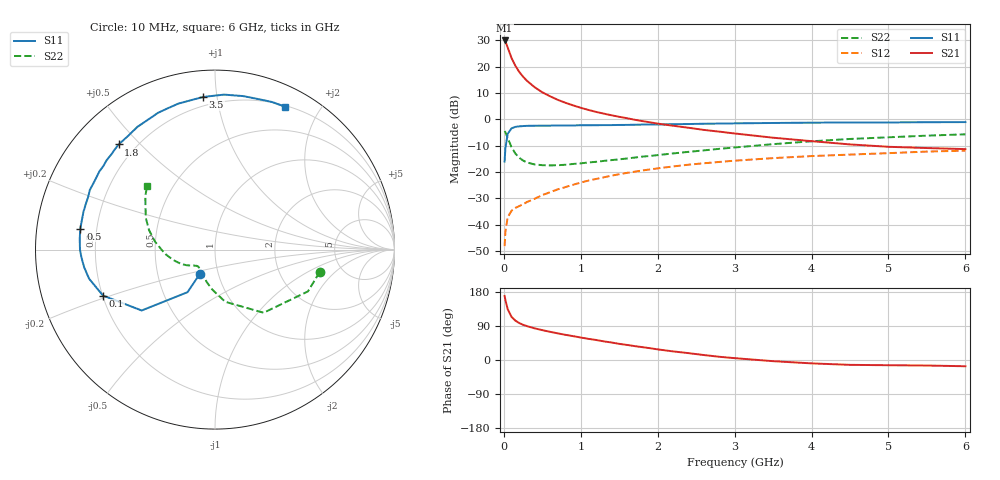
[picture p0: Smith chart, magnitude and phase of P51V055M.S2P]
! SIEMENS Small Signal Semiconductors
! BFP183
! Si NPN RF Bipolar Junction Transistor in SOT143
! VCE = 1 V  IC = 55 mA
! Common Emitter S-Parameters:  March  1996
# GHz  S  MA  R  50
!  f  S11  S21  S12  S22
! GHz  MAG  ANG  MAG  ANG  MAG  ANG  MAG  ANG
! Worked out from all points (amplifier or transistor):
!   36 points, 10 MHz to 6 GHz, reference 50 ohm
!   highest |S21| = 30.0 dB at 10 MHz (marker M1)
!   |S21| within 3 dB of that: start of sweep to 54.15 MHz
!   unconditionally stable (mu >= 1): start of sweep to 36.99 MHz; 132.7 MHz to end of sweep
!   at 250 MHz: K = 1.40, MAG = 20.5 dB, |S12| = -32.3 dB
!   at 1.4 GHz: K = 1.98, MAG = 5.8 dB, |S12| = -21.4 dB
!   at 6 GHz: K = 1.56, MAG = -4.1 dB, |S12| = -11.9 dB
!   S11 on the Smith chart (normalised r, x): 10 MHz: 0.82, -0.23; 100 MHz: 0.20, -0.19; 500 MHz: 0.14, +0.08; 1.8 GHz: 0.14, +0.43; 3.5 GHz: 0.15, +0.91; 6 GHz: 0.21, +1.58
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0.01  0.158 -121.9  31.5 169.0  0.0039 64.1  0.5965 -12.1
0.02  0.2823 -122.8  30.21 158.4  0.0074 60.8  0.5679 -24.2
0.05  0.5311 -140.3  23.17 134.2  0.0138 51.6  0.444 -52.4
0.1  0.6747 -157.7  14.62 113.9  0.0183 40.7  0.2963 -78.9
0.15  0.7202 -167.0  10.4 103.9  0.0208 40.5  0.2236 -93.8
0.2  0.7355 -172.3  7.962 97.5  0.0225 42.5  0.1868 -104.2
0.25  0.7457 -176.8  6.455 92.9  0.0244 45.0  0.1651 -111.7
0.3  0.7522 -179.9  5.407 89.4  0.0269 47.5  0.1517 -117.4
0.4  0.7562 175.4  4.076 83.6  0.031 52.5  0.1392 -125.5
0.5  0.7594 171.1  3.263 78.8  0.0364 54.4  0.1347 -131.0
0.6  0.7596 167.5  2.745 74.4  0.0413 56.7  0.1334 -134.4
0.7  0.7624 164.1  2.348 70.3  0.0467 58.3  0.1345 -137.0
0.9  0.7648 157.7  1.842 63.0  0.0572 59.0  0.1421 -140.6
1.1  0.7716 151.5  1.508 55.8  0.0687 58.9  0.1515 -144.1
1.5  0.7827 140.5  1.117 42.6  0.0907 56.4  0.1738 -149.8
1.8  0.7948 132.5  0.927 33.9  0.1068 53.7  0.1959 -155.1
2.2  0.8089 122.4  0.756 22.7  0.1274 49.1  0.2252 -162.7
2.8  0.8305 108.2  0.584 8.5  0.1552 41.5  0.2752 -174.4
3.5  0.8529 94.5  0.448 -3.1  0.1834 33.2  0.3379 172.3
4.5  0.8695 79.6  0.334 -12.8  0.2141 21.6  0.424 155.4
5.5  0.8817 68.8  0.285 -14.6  0.2442 11.6  0.4902 142.4
6  0.8863 63.9  0.272 -16.5  0.2543 6.3  0.5192 136.6
